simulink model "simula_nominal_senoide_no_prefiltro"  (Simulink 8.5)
settings: Solver=ode45  StartTime=0.0  StopTime=tf  RelTol=1e-3
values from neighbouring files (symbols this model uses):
  denF = [1 qsi2wn wn2]    [princi_JL_incerto_prefilt_2a_ordem.m]
  denK = [1/6 1]    [princi_JL_incerto_prefilt_2a_ordem.m]
  knom = r*kT/Ra/Jeq    [princi_JL_incerto_prefilt_2a_ordem.m]
  numF = [wn2]    [princi_JL_incerto_prefilt_2a_ordem.m]
  numK = 2.5    [princi_JL_incerto_prefilt_2a_ordem.m]
  pnom = feq/Jeq    [princi_JL_incerto_prefilt_2a_ordem.m]
  w0_pre_filt = wF    (= 0.36)    [princi_JL_incerto_prefilt_2a_ordem.m]

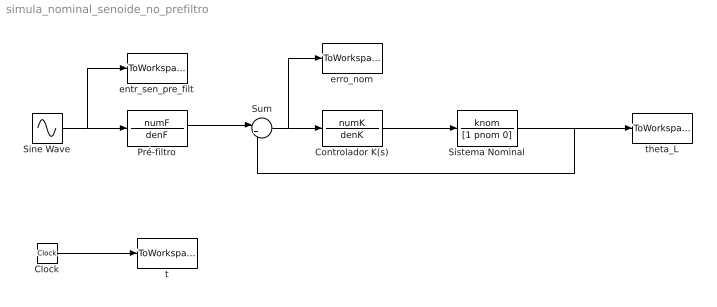
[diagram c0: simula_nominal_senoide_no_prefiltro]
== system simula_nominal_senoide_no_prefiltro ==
  Clock : Clock
  Controlador K(s) : TransferFcn  Numerator=numK  Denominator=denK
  Pré-filtro : TransferFcn  Numerator=numF  Denominator=denF
  Sine Wave : Sin  Frequency=w0_pre_filt  SampleTime=0
  Sistema Nominal : TransferFcn  Numerator=knom  Denominator=[1 pnom 0]
  Sum : Sum  Inputs=|+-
  entr_sen_pre_filt : ToWorkspace  VariableName=entr_sen_pre_filt  SampleTime=-1
  erro_nom : ToWorkspace  VariableName=erro_nom  SampleTime=-1
  t : ToWorkspace  VariableName=t  SampleTime=-1
  theta_L : ToWorkspace  VariableName=theta_L_nom  SampleTime=-1
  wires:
  Sum/1 -> erro_nom/1, Controlador K(s)/1
  Pré-filtro/1 -> Sum/1
  Clock/1 -> t/1
  Controlador K(s)/1 -> Sistema Nominal/1
  Sistema Nominal/1 -> Sum/2, theta_L/1
  Sine Wave/1 -> entr_sen_pre_filt/1, Pré-filtro/1
